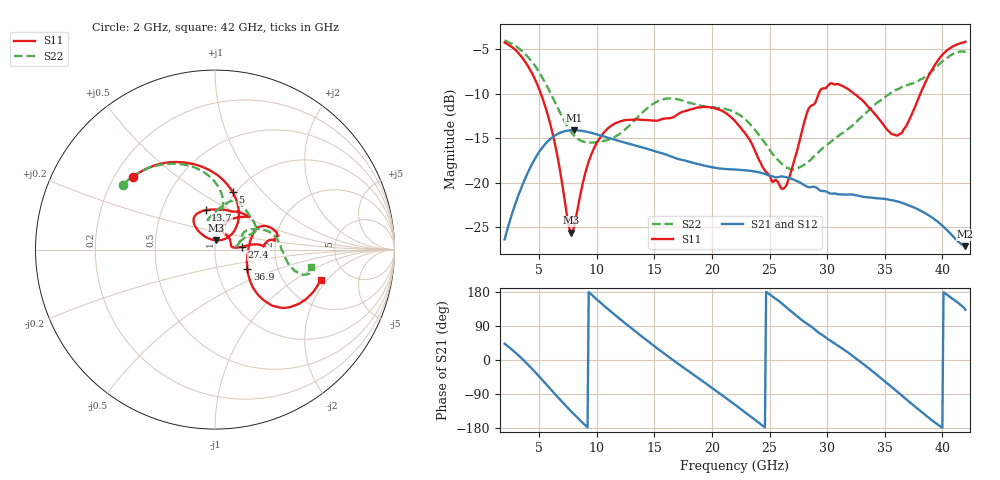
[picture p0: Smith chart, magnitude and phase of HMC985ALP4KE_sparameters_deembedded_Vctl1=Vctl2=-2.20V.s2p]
!s2p File: Measurements: S11, S21, S12, S22
# GHz S dB R 50.0
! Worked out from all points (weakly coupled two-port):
!   401 points, 2 GHz to 42 GHz, reference 50 ohm
!   highest |S21| = -14.12 dB at 8 GHz (marker M1); lowest = -27.1 dB at 42 GHz (marker M2)
!   lowest |S11| = -25.6 dB at 7.8 GHz (marker M3), VSWR 1.11, Z = 50.2 + j5.23 ohm
!   |S11| at or under -10 dB: 5.142 GHz to 29.27 GHz (24.13 GHz wide, 140 % of centre); 32.31 GHz to 38.1 GHz (5.788 GHz wide, 16.4 % of centre)
!   |S22| runs from -18.5 to -4.0 dB; largest |S21 - S12| = 0.00021
!   S11 on the Smith chart (normalised r, x): 2 GHz: 0.27, +0.35; 5 GHz: 0.97, +0.70; 13.7 GHz: 0.82, +0.38; 27.4 GHz: 1.35, +0.04; 36.9 GHz: 1.40, -0.32; 42 GHz: 3.18, -1.76
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2  -4.27 138.5  -26.39 43.1  -26.40 43.1  -4.04 144.9
3.5  -5.93 107.3  -20.43 3.7  -20.44 3.7  -5.22 119.5
5  -9.51 72.9  -16.56 -43.5  -16.57 -43.5  -7.61 95.4
6.2  -14.68 48.1  -14.86 -84.0  -14.87 -84.0  -10.51 82.1
7.8  -25.65 84.5  -14.13 -136.3  -14.13 -136.3  -14.37 84.4
8  -25.13 101.2  -14.12 -142.5  -14.12 -142.5  -14.69 86.4
8.7  -20.58 128.0  -14.19 -163.5  -14.20 -163.5  -15.36 94.0
10.6  -14.41 128.2  -14.81 144.0  -14.82 144.0  -15.34 103.8
13.7  -12.95 103.3  -15.97 67.2  -15.97 67.2  -12.46 82.3
15.4  -13.00 81.8  -16.63 27.3  -16.62 27.3  -10.82 70.8
19  -11.57 44.9  -18.00 -51.6  -18.01 -51.7  -11.37 44.6
22  -13.09 54.1  -18.54 -118.0  -18.55 -118.1  -12.11 24.1
24.5  -18.45 74.4  -18.99 -175.4  -18.99 -175.4  -15.38 20.9
26.1  -20.72 16.2  -19.32 148.3  -19.32 148.3  -17.95 12.4
27.4  -16.38 6.0  -19.84 115.2  -19.84 115.1  -18.44 8.3
28.7  -11.31 3.6  -20.48 86.4  -20.50 86.3  -17.25 14.2
31.1  -9.03 16.3  -21.33 34.7  -21.34 34.6  -14.65 30.5
33.3  -11.10 27.1  -21.64 -14.5  -21.64 -14.5  -12.28 27.8
35.4  -14.30 7.5  -21.92 -66.2  -21.91 -66.2  -10.07 18.8
36.9  -13.56 -31.0  -22.47 -104.5  -22.47 -104.4  -9.07 9.5
39.7  -6.12 -41.0  -24.51 -172.5  -24.51 -172.6  -6.77 -15.0
42  -4.19 -16.1  -27.15 132.7  -27.14 132.6  -5.28 -10.4
